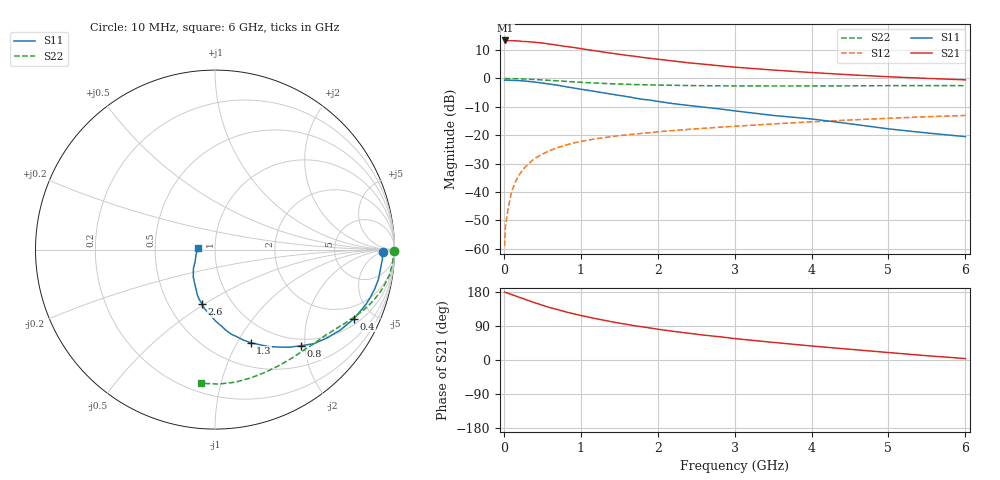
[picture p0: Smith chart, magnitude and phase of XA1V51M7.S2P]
! SIEMENS Discrete & RF Semiconductors
! BFY180
! Si NPN RF Bipolar Junction Transistor in MICRO-X
! VCE = 1.5 V  IC = 1.7 mA
! Common Emitter S-Parameters:  May  1997
# GHz  S  MA  R  50
!  f  S11  S21  S12  S22
! GHz  MAG  ANG  MAG  ANG  MAG  ANG  MAG  ANG
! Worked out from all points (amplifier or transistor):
!   36 points, 10 MHz to 6 GHz, reference 50 ohm
!   highest |S21| = 13.4 dB at 20 MHz (marker M1)
!   |S21| within 3 dB of that: start of sweep to 1.031 GHz
!   unconditionally stable (mu >= 1): 2.497 GHz to end of sweep
!   at 250 MHz: K = 0.14, MSG = 22.6 dB, |S12| = -32.0 dB
!   at 1.4 GHz: K = 0.72, MSG = 14.7 dB, |S12| = -20.5 dB
!   at 6 GHz: K = 1.11, MAG = 4.3 dB, |S12| = -13.0 dB
!   S11 on the Smith chart (normalised r, x): 10 MHz: 29, -5; 400 MHz: 1.27, -3.87; 800 MHz: 0.87, -1.92; 1.3 GHz: 0.76, -1.14; 2.6 GHz: 0.73, -0.49; 6 GHz: 0.83, +0.01
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0.01  0.9343 -0.7  4.627 179.3  0.0011 93.4  0.9951 -0.3
0.02  0.9327 -1.6  4.69 178.4  0.0024 86.4  0.9999 -0.6
0.05  0.9343 -3.2  4.647 176.5  0.0046 86.8  0.9945 -1.6
0.1  0.9281 -6.7  4.645 172.8  0.01 85.9  0.9932 -3.4
0.15  0.9256 -10.2  4.628 169.2  0.015 85.4  0.9908 -5.0
0.25  0.9062 -16.9  4.5 162.1  0.025 79.3  0.9828 -8.3
0.3  0.8947 -20.0  4.477 158.2  0.0294 76.8  0.9744 -9.7
0.4  0.865 -26.4  4.358 151.2  0.0387 73.3  0.961 -12.7
0.5  0.8308 -32.5  4.224 144.6  0.0463 69.7  0.9432 -15.5
0.6  0.7966 -38.0  4.047 138.1  0.0536 66.0  0.926 -17.9
0.8  0.7184 -48.2  3.678 127.1  0.0665 60.5  0.8914 -22.4
0.9  0.683 -52.8  3.54 122.3  0.0725 57.8  0.8734 -24.5
1.1  0.6167 -61.2  3.205 113.3  0.0819 53.9  0.8432 -28.0
1.3  0.5553 -69.1  2.92 105.1  0.0903 50.4  0.8181 -31.3
1.5  0.5031 -75.6  2.676 97.3  0.0983 47.8  0.7982 -34.3
1.7  0.4537 -82.3  2.469 90.4  0.1044 45.9  0.7816 -37.1
2.2  0.3603 -94.7  2.038 75.7  0.1207 41.4  0.7591 -44.1
2.6  0.3119 -103.3  1.787 65.6  0.1322 38.4  0.7464 -49.3
3.5  0.2231 -120.2  1.41 46.5  0.1579 32.3  0.7379 -61.0
4.5  0.1589 -139.0  1.163 28.3  0.1852 25.1  0.7421 -74.4
5.5  0.1094 -165.2  1.005 11.3  0.2114 17.2  0.7493 -88.6
6  0.0942 175.0  0.946 3.8  0.2228 12.9  0.7488 -95.8
